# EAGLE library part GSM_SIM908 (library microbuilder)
SIM908 GSM + GPS Module
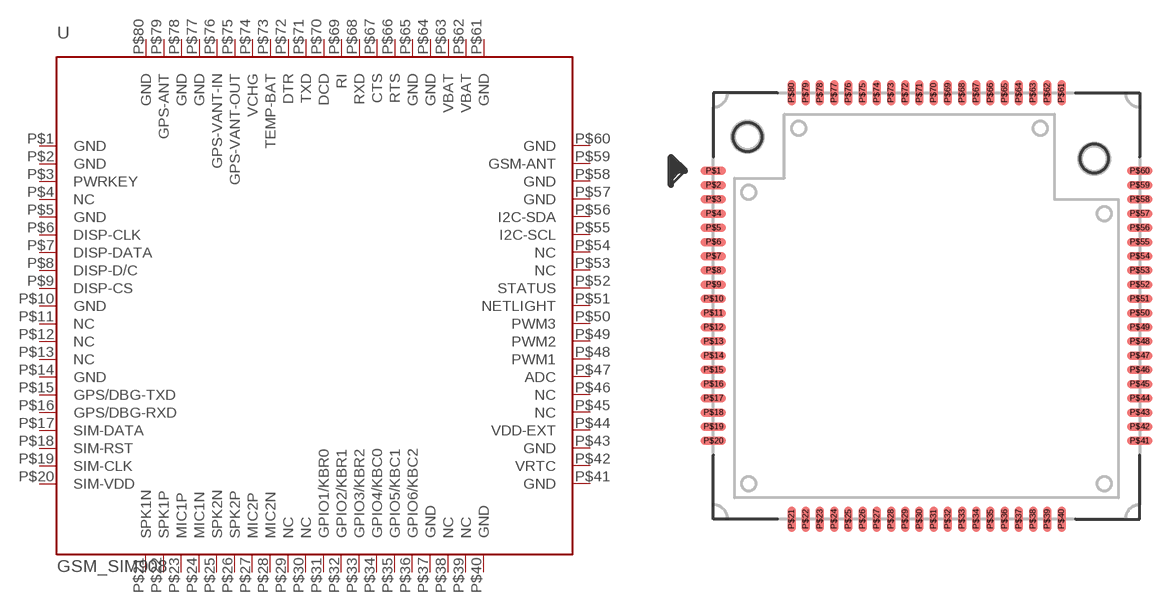
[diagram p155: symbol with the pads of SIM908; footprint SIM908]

Designator prefix U

## GSM_SIM908  [SIM908]
P$1  GND  pwr
P$2  GND  pwr
P$3  PWRKEY  in
P$4  NC  nc
P$5  GND  pwr
P$6  DISP-CLK  out
P$7  DISP-DATA
P$8  DISP-D/C  out
P$9  DISP-CS  out
P$10  GND  pwr
P$11  NC  nc
P$12  NC  nc
P$13  NC  nc
P$14  GND  pwr
P$15  GPS/DBG-TXD  out
P$16  GPS/DBG-RXD  in
P$17  SIM-DATA
P$18  SIM-RST  out
P$19  SIM-CLK  out
P$20  SIM-VDD  pwr
P$21  SPK1N  out
P$22  SPK1P  out
P$23  MIC1P  in
P$24  MIC1N  in
P$25  SPK2N  out
P$26  SPK2P  out
P$27  MIC2P  in
P$28  MIC2N  in
P$29  NC  nc
P$30  NC  nc
P$31  GPIO1/KBR0
P$32  GPIO2/KBR1
P$33  GPIO3/KBR2
P$34  GPIO4/KBC0
P$35  GPIO5/KBC1
P$36  GPIO6/KBC2
P$37  GND  pwr
P$38  NC  nc
P$39  NC  nc
P$40  GND  pwr
P$41  GND  pwr
P$42  VRTC  pwr
P$43  GND  pwr
P$44  VDD-EXT  pwr
P$45  NC  nc
P$46  NC  nc
P$47  ADC  in
P$48  PWM1  out
P$49  PWM2  out
P$50  PWM3  out
P$51  NETLIGHT  out
P$52  STATUS  out
P$53  NC  nc
P$54  NC  nc
P$55  I2C-SCL
P$56  I2C-SDA  out
P$57  GND  pwr
P$58  GND  pwr
P$59  GSM-ANT
P$60  GND  pwr
P$61  GND  pwr
P$62  VBAT  pwr
P$63  VBAT  pwr
P$64  GND  pwr
P$65  GND  pwr
P$66  RTS  out
P$67  CTS  in
P$68  RXD  in
P$69  RI  out
P$70  DCD  out
P$71  TXD  out
P$72  DTR  in
P$73  TEMP-BAT  in
P$74  VCHG  pwr
P$75  GPS-VANT-OUT  pwr
P$76  GPS-VANT-IN  pwr
P$77  GND  pwr
P$78  GND  pwr
P$79  GPS-ANT  in
P$80  GND  pwr

## Footprint SIM908 (pad centres in mm)
smd 1.8 x 0.6: P$1 -15,9.5; P$2 -15,8.5; P$3 -15,7.5; P$4 -15,6.5; P$5 -15,5.5; P$6 -15,4.5; P$7 -15,3.5; P$8 -15,2.5; P$9 -15,1.5; P$10 -15,0.5; P$11 -15,-0.5; P$12 -15,-1.5; P$13 -15,-2.5; P$14 -15,-3.5; P$15 -15,-4.5; P$16 -15,-5.5; P$17 -15,-6.5; P$18 -15,-7.5; P$19 -15,-8.5; P$20 -15,-9.5; P$41 15,-9.5; P$42 15,-8.5; P$43 15,-7.5; P$44 15,-6.5; P$45 15,-5.5; P$46 15,-4.5; P$47 15,-3.5; P$48 15,-2.5; P$49 15,-1.5; P$50 15,-0.5; P$51 15,0.5; P$52 15,1.5; P$53 15,2.5; P$54 15,3.5; P$55 15,4.5; P$56 15,5.5; P$57 15,6.5; P$58 15,7.5; P$59 15,8.5; P$60 15,9.5
smd 0.6 x 1.8: P$21 -9.5,-15; P$22 -8.5,-15; P$23 -7.5,-15; P$24 -6.5,-15; P$25 -5.5,-15; P$26 -4.5,-15; P$27 -3.5,-15; P$28 -2.5,-15; P$29 -1.5,-15; P$30 -0.5,-15; P$31 0.5,-15; P$32 1.5,-15; P$33 2.5,-15; P$34 3.5,-15; P$35 4.5,-15; P$36 5.5,-15; P$37 6.5,-15; P$38 7.5,-15; P$39 8.5,-15; P$40 9.5,-15; P$61 9.5,15; P$62 8.5,15; P$63 7.5,15; P$64 6.5,15; P$65 5.5,15; P$66 4.5,15; P$67 3.5,15; P$68 2.5,15; P$69 1.5,15; P$70 0.5,15; P$71 -0.5,15; P$72 -1.5,15; P$73 -2.5,15; P$74 -3.5,15; P$75 -4.5,15; P$76 -5.5,15; P$77 -6.5,15; P$78 -7.5,15; P$79 -8.5,15; P$80 -9.5,15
